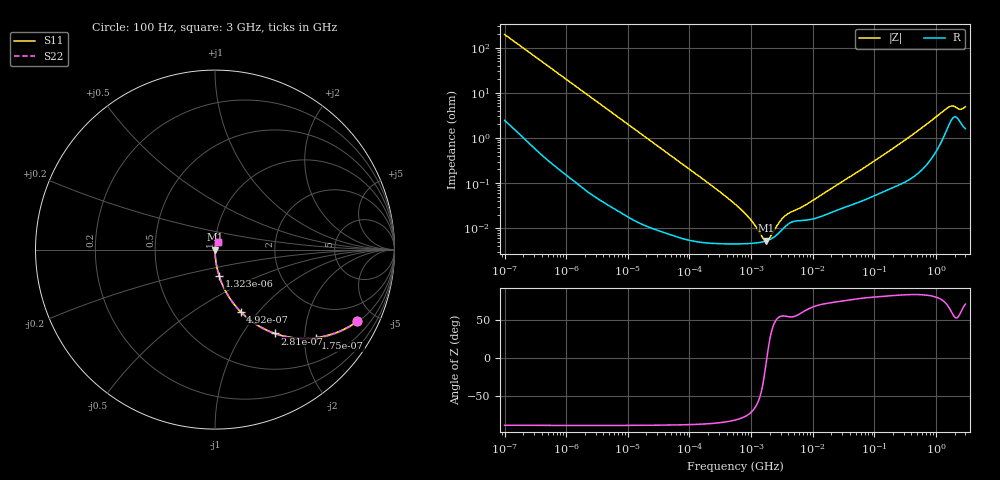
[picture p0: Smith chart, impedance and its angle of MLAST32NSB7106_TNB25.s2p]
! MLAST32NSB7106_TNB25  S-PARAMETER MODEL  ( Standard Model )
! Model Generated by TAIYO YUDEN Corporation (http://www.ty-top.com)
! Version 2.0
! TAIYO YUDEN Control No. 240510
! Copyright(c) 2011 TAIYO YUDEN CO.,LTD. All Rights Reserved.
! Product Description (link to TY-COMPAS)
! https://ds.yuden.co.jp/TYCOMPAS/or/detail?pn=MLAST32NSB7106KTNB25&u=M
! Products Name : Multilayer Ceramic Capacitors
! Characteristics :
!  Capacitance : 10 [uF] , Rated Voltage : 25 [V] , TCC : X7R
!  Case Size : 3.2 x 2.5 / 0.126 x 0.098 [mm/inch] , Thickness : 1.9 / 0.075 [mm/inch]
!  (Conditions: Temperature = 25 [degC] , DC Bias Voltage = 0 [V])
! External Node Assignments :
!  1  o---| |---o  2
! GND o---------o GND
! Frequency Range : 100Hz  -  3GHz  [ 401 STEP ]
# MHZ S RI R 50
! Freq[MHz].  S11 Real  S11 Imag  S21 Real  S21 Imag  S12 Real  S12 Imag  S22 Real  S22 Imag
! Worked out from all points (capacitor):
!   401 points, 100 Hz to 3 GHz, reference 50 ohm
!   read as one part in series: C = 8.06 uF near 109 Hz
!   lowest |Z| = 5.24 mohm at 1.751 MHz (marker M1)
!   series resonance near 1.803 MHz, so ESL is about 970 pH
!   S11 on the Smith chart (normalised r, x): 100 Hz: 1.05, -3.94; 175 Hz: 1.02, -2.26; 281 Hz: 1.01, -1.41; 492 Hz: 1.01, -0.81; 1.323 kHz: 1.00, -0.30; 3 GHz: 1.03, +0.09
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0.0001  0.7922 -0.3995  0.2078 0.3995  0.2078 0.3995  0.7922 -0.3995
0.000175  0.5606 -0.491  0.4394 0.491  0.4394 0.491  0.5606 -0.491
0.000281  0.3344 -0.4672  0.6656 0.4672  0.6656 0.4672  0.3344 -0.4672
0.000492  0.1428 -0.3458  0.8572 0.3458  0.8572 0.3458  0.1428 -0.3458
0.000756  0.0667 -0.2456  0.9333 0.2456  0.9333 0.2456  0.0667 -0.2456
0.001323  0.0233 -0.1474  0.9767 0.1474  0.9767 0.1474  0.0233 -0.1474
0.001788  0.0131 -0.1103  0.9869 0.1103  0.9869 0.1103  0.0131 -0.1103
0.005476  0.00163 -0.0366  0.9984 0.0366  0.9984 0.0366  0.00163 -0.0366
0.031977  0.000127 -0.00633  0.9999 0.00633  0.9999 0.00633  0.000127 -0.00633
0.221826  4.7e-05 -0.000906  1 0.000906  1 0.000906  4.7e-05 -0.000906
0.547723  4.48e-05 -0.000339  1 0.000339  1 0.000339  4.48e-05 -0.000339
0.806856  4.52e-05 -0.000204  1 0.000204  1 0.000204  4.52e-05 -0.000204
1.240863  4.71e-05 -8.8e-05  1 8.8e-05  1 8.8e-05  4.71e-05 -8.8e-05
1.75092  5.2e-05 -6.82e-06  0.9999 6.82e-06  0.9999 6.82e-06  5.2e-05 -6.82e-06
2.366551  6.38e-05 6.41e-05  0.9999 -6.41e-05  0.9999 -6.41e-05  6.38e-05 6.41e-05
3.79959  0.000116 0.000164  0.9999 -0.000164  0.9999 -0.000164  0.000116 0.000164
9.794414  0.000159 0.00037  0.9998 -0.00037  0.9998 -0.00037  0.000159 0.00037
175.1444  0.000757 0.00511  0.9992 -0.00511  0.9992 -0.00511  0.000757 0.00511
1573.002  0.0192 0.0424  0.9808 -0.0424  0.9808 -0.0424  0.0192 0.0424
1868.531  0.0285 0.0409  0.9715 -0.0409  0.9715 -0.0409  0.0285 0.0409
2525.516  0.0223 0.0359  0.9777 -0.0359  0.9777 -0.0359  0.0223 0.0359
3000  0.0179 0.0451  0.9821 -0.0451  0.9821 -0.0451  0.0179 0.0451
